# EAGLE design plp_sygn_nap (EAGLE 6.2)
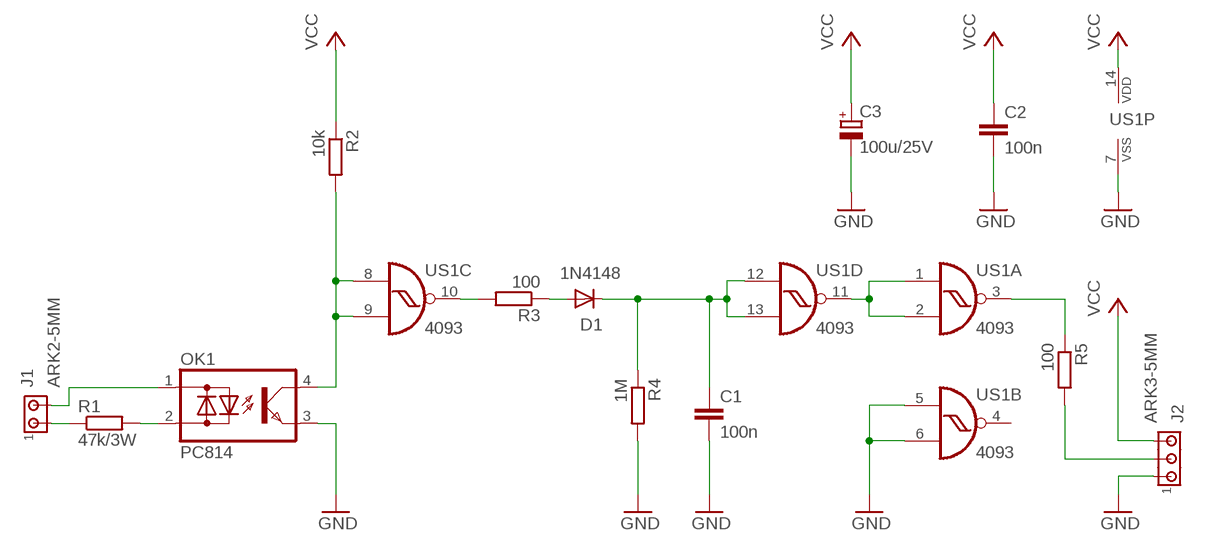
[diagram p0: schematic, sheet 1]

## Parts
C1  100n  C-EU050-025X075  [C050-025X075]
C2  100n  C-EU050-025X075  [C050-025X075]
C3  100u/25V  CPOL-EUE2.5-6  [E2,5-6]
D1  1N4148  1N4148DO35-7  [DO35-7]
J1  ARK2-5MM  [2PIN-5MM]
J2  ARK3-5MM  [3PIN-5MM]
OK1  PC814  [DIL04]
R1  47k/3W  R-EU_0617/17  [0617/17]
R2  10k  R-EU_0207/7  [0207/7]
R3  100  R-EU_0207/7  [0207/7]
R4  1M  R-EU_0207/7  [0207/7]
R5  100  R-EU_0207/7  [0207/7]
US1  4093  4093N  [DIL14]

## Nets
GND: C1.2 C2.2 C3.- J2.P$1 OK1.3(E) R4.2 US1.5(B:I0) US1.6(B:I1) US1.7(P:VSS)
N$1: J1.P$1 R1.1
N$2: OK1.2(AC2) R1.2
N$3: J1.P$2 OK1.1(AC1)
N$5: OK1.4(C) R2.2 US1.8(C:I0) US1.9(C:I1)
N$6: R3.2 US1.10(C:O)
N$7: R5.1 US1.3(A:O)
N$8: D1.A R3.1
N$9: J2.P$2 R5.2
N$10: US1.1(A:I0) US1.2(A:I1) US1.11(D:O)
N$12: C1.1 D1.C R4.1 US1.12(D:I0) US1.13(D:I1)
VCC: C2.1 C3.+ J2.P$3 R2.1 US1.14(P:VDD)
Unconnected: US1.4(B:O)

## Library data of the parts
C1 C2 = rcl:C-EU: CAPACITOR, European symbol
C3 = rcl:CPOL-EU: POLARIZED CAPACITOR, European symbol
D1 = diode:1N4148: DIODE
J1 = zlacza_futrzak:ARK2: ARK 2
J2 = zlacza_futrzak:ARK3: ARK 3 Raster 5mm i 3,5mm
OK1 = optocoupler:PC814: SHARP OPTO COUPLER; OC_FARNELL: 9707662; OC_NEWARK: unknown
R1-R5 = rcl:R-EU_: RESISTOR, European symbol
US1 = 40xx:4093: Quad 2-input NAND schmitt trigger

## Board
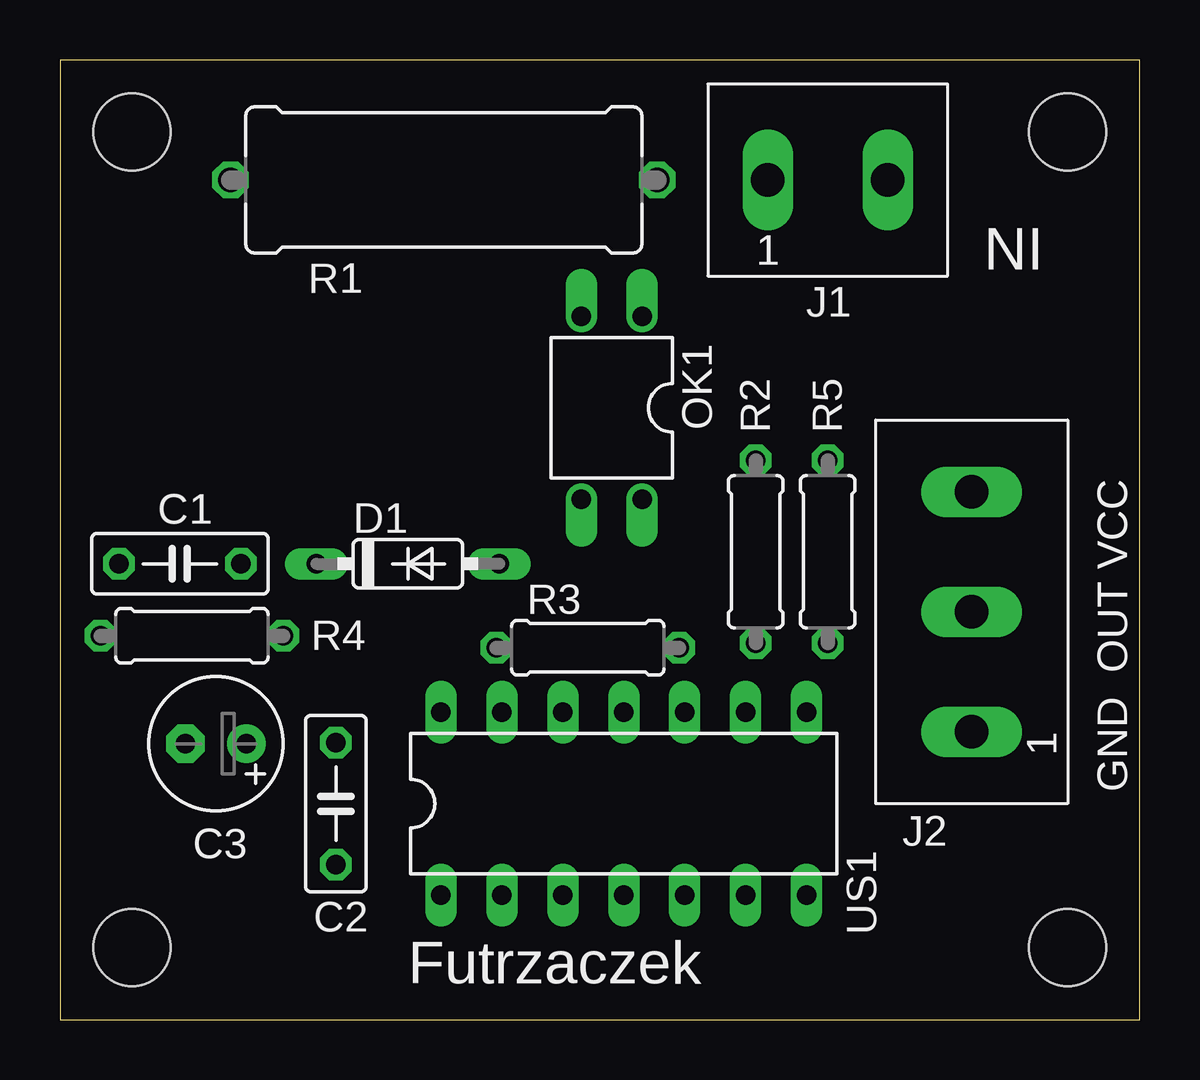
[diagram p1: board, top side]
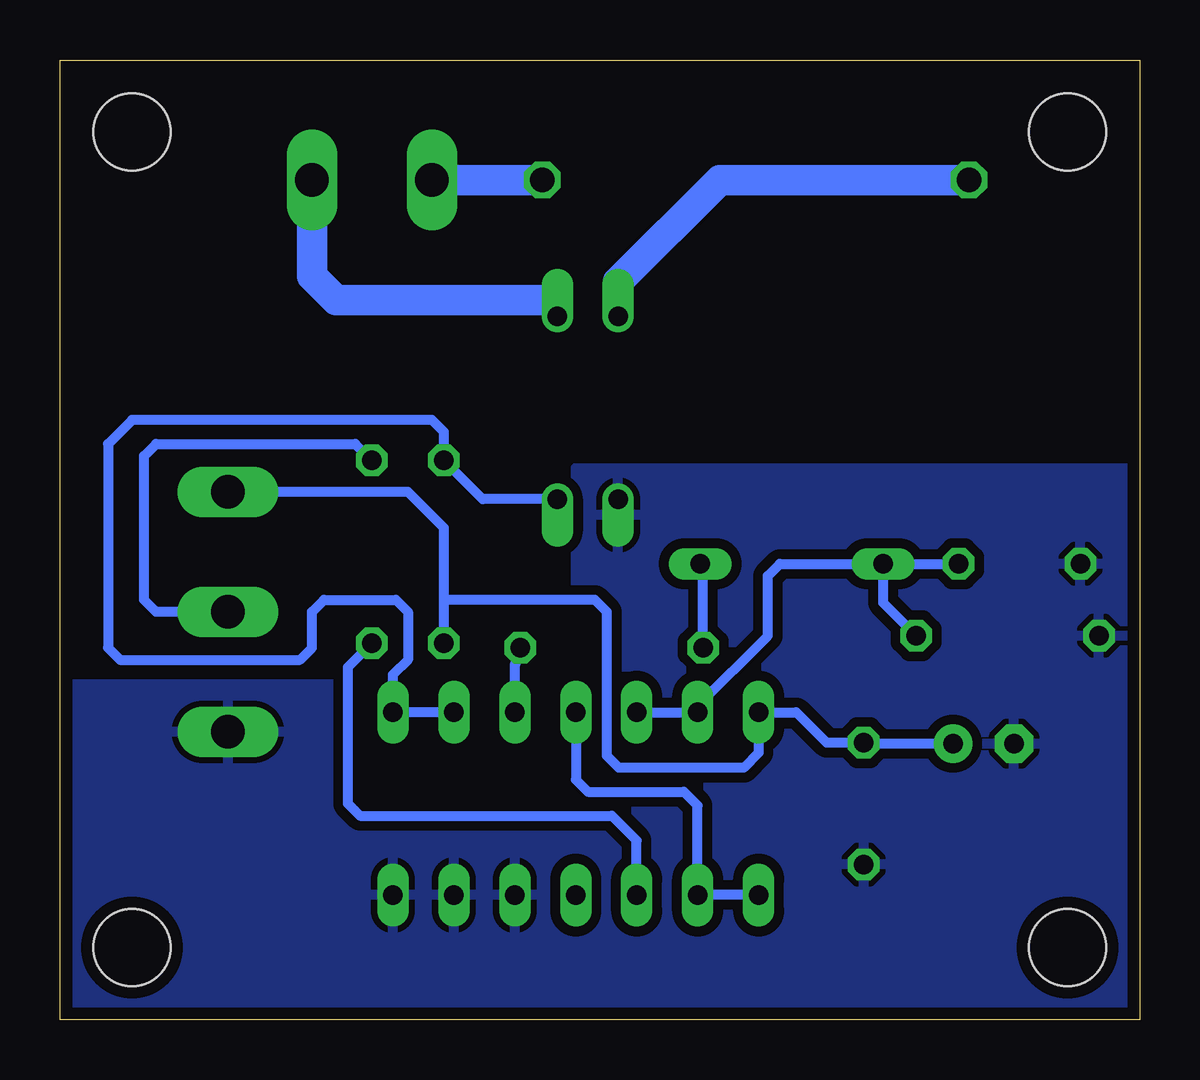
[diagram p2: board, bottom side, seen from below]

Size 45 x 40 mm. Coordinates in mm from the lower left corner, seen from the top.
Outline: 0,0 45,0 45,40 0,40 0,0
Copper layers (1*16): Top 0.035mm / dielectric 1.5mm / Bottom 0.035mm
Design rules: minimum track width 10mil, minimum drill 24mil, track to track 8mil, track to pad 8mil, pad to pad 8mil, via to via 8mil, smd to smd 8mil, copper to edge 20mil, drill to drill 8mil, minimum pad ring 10mil, minimum via ring 8mil, stop-mask expansion 4mil, vias tented up to drill 0mil, thermal gap 10mil
Holes 3.2 mm at 3,37 42,37 3,3 42,3

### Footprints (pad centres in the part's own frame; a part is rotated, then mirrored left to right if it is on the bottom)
C050-025X075 = drill 0.813 octagon: 1 -2.54,0; 2 2.54,0
E2,5-6 = drill 0.813 pad 1.6: + -1.27,0 | drill 0.813 pad 1.6 octagon: - 1.27,0
DO35-7 = drill 0.813 long: A 3.81,0; C -3.81,0
2PIN-5MM = drill 1.4 long: P$1 -2.5,0; P$2 2.5,0
3PIN-5MM = drill 1.4 long: P$1 -5,0; P$2 0,0; P$3 5,0
DIL04 = drill 0.813 offset: 1 -1.27,-3.81; 2 1.27,-3.81; 3 1.27,3.81; 4 -1.27,3.81
0617/17 = drill 1.016 octagon: 1 -8.89,0; 2 8.89,0
0207/7 = drill 0.813 octagon: 1 -3.81,0; 2 3.81,0
DIL14 = drill 0.813 long: 1 -7.62,-3.81; 2 -5.08,-3.81; 3 -2.54,-3.81; 4 0,-3.81; 5 2.54,-3.81; 6 5.08,-3.81; 7 7.62,-3.81; 8 7.62,3.81; 9 5.08,3.81; 10 2.54,3.81; 11 0,3.81; 12 -2.54,3.81; 13 -5.08,3.81; 14 -7.62,3.81

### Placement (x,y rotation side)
C1  5,19 180 top
C2  11.5,9 270 top
C3  6.5,11.5 180 top
D1  14.5,19 0 top
J1  32,35 0 top
J2  38,17 90 top
OK1  23,25.5 180 top
R1  16,35 180 top
R2  29,19.5 90 top
R3  22,15.5 0 top
R4  5.5,16 180 top
R5  32,19.5 90 top
US1  23.5,9 0 top

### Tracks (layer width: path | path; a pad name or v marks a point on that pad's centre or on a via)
GND
  pour Bottom (isolate 0.406): 0,0 45,0 45,14 23.5,14 23.5,23 0,23
N$1
  Bottom 1.27: J1.P$1 R1.1
N$2
  Bottom 1.27: OK1.2 21.73,30.77 17.5,35 R1.2
N$3
  Bottom 1.27: OK1.1 24.27,30.27 24.5,30 33.5,30 34.5,31 J1.P$2
N$5
  Bottom 0.406: US1.9 US1.8 31.12,14.38 30.5,15 30.5,17 31,17.5 34,17.5 34.5,17 34.5,15.5 35,15 42.5,15 43,15.5 43,24 42,25 29.5,25 29,24.5 R2.2 27.38,21.69 OK1.4
N$6
  Bottom 0.406: US1.10 26.04,14.77 R3.2
N$7
  Bottom 0.406: R5.1 33,14.69 33,9 32.5,8.5 22,8.5 20.96,7.46 US1.3
N$8
  Bottom 0.406: R3.1 18.19,18.88 D1.A
N$9
  Bottom 0.406: J2.P$2 41,17 41.5,17.5 41.5,23.5 41,24 32.69,24 R5.2
N$10
  Bottom 0.406: US1.11 23.5,10 23,9.5 19,9.5 18.42,8.92 US1.2 US1.1
N$12
  Bottom 0.406: US1.12 US1.13 18.42,13.08 15.5,16 15.5,18.5 15,19 D1.C | D1.C C1.1 | D1.C 10.69,17.38 R4.1
VCC
  Bottom 0.406: R2.1 29,17.5 | 29,17.5 29,20.5 30.5,22 J2.P$3 | C3.+ 11.46,11.5 C2.1 13.04,11.54 14.31,12.81 US1.14 15.88,11.12 16.5,10.5 21.7,10.5 22.2,11 22.2,17 22.7,17.5 29,17.5

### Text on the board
tPlace: IN | GND OUT VCC | Futrzaczek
